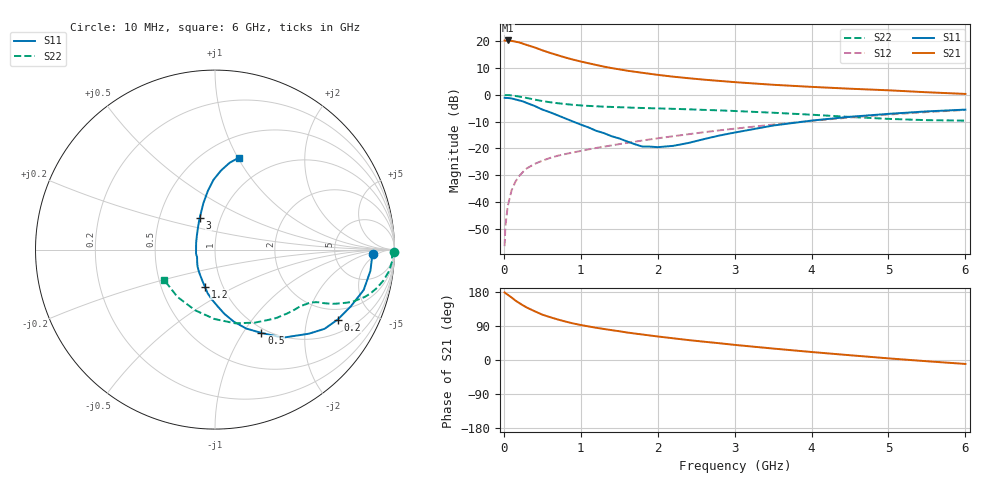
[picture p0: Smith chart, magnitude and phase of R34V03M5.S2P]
! SIEMENS Small Signal Semiconductors
! BFR181
! Si NPN RF Bipolar Junction Transistor in SOT23
! VCE = 4 V  IC = 3.5 mA
! Common Emitter S-Parameters:  May  1996
# GHz  S  MA  R  50
!  f  S11  S21  S12  S22
! GHz  MAG  ANG  MAG  ANG  MAG  ANG  MAG  ANG
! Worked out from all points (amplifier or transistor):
!   36 points, 10 MHz to 6 GHz, reference 50 ohm
!   highest |S21| = 20.3 dB at 50 MHz (marker M1)
!   |S21| within 3 dB of that: start of sweep to 437.5 MHz
!   unconditionally stable (mu >= 1): 1.293 GHz to 3.144 GHz
!   at 250 MHz: K = 0.33, MSG = 23.9 dB, |S12| = -28.7 dB
!   at 1.4 GHz: K = 1.02, MAG = 13.5 dB, |S12| = -18.9 dB
!   at 6 GHz: K = 0.86, MSG = 3.0 dB, |S12| = -5.6 dB
!   S11 on the Smith chart (normalised r, x): 10 MHz: 15, -3; 200 MHz: 1.51, -3.09; 500 MHz: 0.94, -1.21; 1.2 GHz: 0.82, -0.36; 3 GHz: 0.80, +0.30; 6 GHz: 0.71, +1.01
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0.01  0.8803 -1.6  10.31 178.3  0.0015 93.5  0.995 -0.7
0.02  0.8761 -2.8  10.19 176.7  0.0035 92.2  0.986 -1.4
0.05  0.8739 -7.8  10.34 172.3  0.0083 89.2  0.9893 -3.7
0.1  0.8584 -15.2  10.15 165.1  0.0164 80.6  0.9767 -7.1
0.15  0.8205 -22.6  9.826 157.0  0.0239 77.3  0.9539 -10.4
0.2  0.7871 -29.7  9.509 150.4  0.0306 73.8  0.9275 -13.3
0.25  0.753 -35.9  8.998 144.1  0.0366 70.7  0.8992 -15.8
0.3  0.7027 -41.8  8.506 138.3  0.0426 68.2  0.8726 -17.7
0.4  0.6202 -52.3  7.672 128.7  0.0514 64.7  0.8152 -21.0
0.5  0.5314 -60.9  6.776 119.7  0.059 62.7  0.7655 -23.0
0.6  0.473 -68.4  6.07 113.1  0.0664 60.8  0.7278 -24.5
0.8  0.3626 -81.6  4.962 101.5  0.0786 59.6  0.6725 -26.3
0.9  0.3172 -87.2  4.541 96.5  0.0842 59.6  0.6512 -26.8
1.1  0.2468 -99.6  3.889 88.7  0.096 60.2  0.6221 -28.2
1.2  0.2136 -105.3  3.609 85.0  0.1019 60.4  0.6111 -28.9
1.6  0.1354 -135.9  2.827 72.6  0.1267 60.7  0.581 -32.2
2.2  0.1116 160.5  2.184 57.3  0.1689 60.6  0.5478 -38.9
3  0.1976 115.4  1.726 39.9  0.2336 57.2  0.4994 -51.0
3.5  0.2672 104.0  1.541 30.2  0.2785 53.9  0.4636 -61.4
4.5  0.3894 91.2  1.301 12.6  0.3777 44.3  0.3868 -90.4
5.5  0.491 80.4  1.117 -3.3  0.4765 31.8  0.3366 -128.5
6  0.5299 75.3  1.04 -10.4  0.522 24.7  0.3303 -149.6
